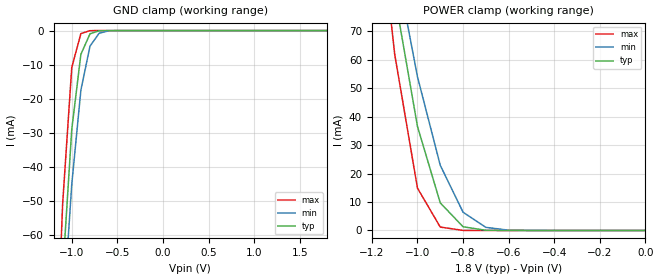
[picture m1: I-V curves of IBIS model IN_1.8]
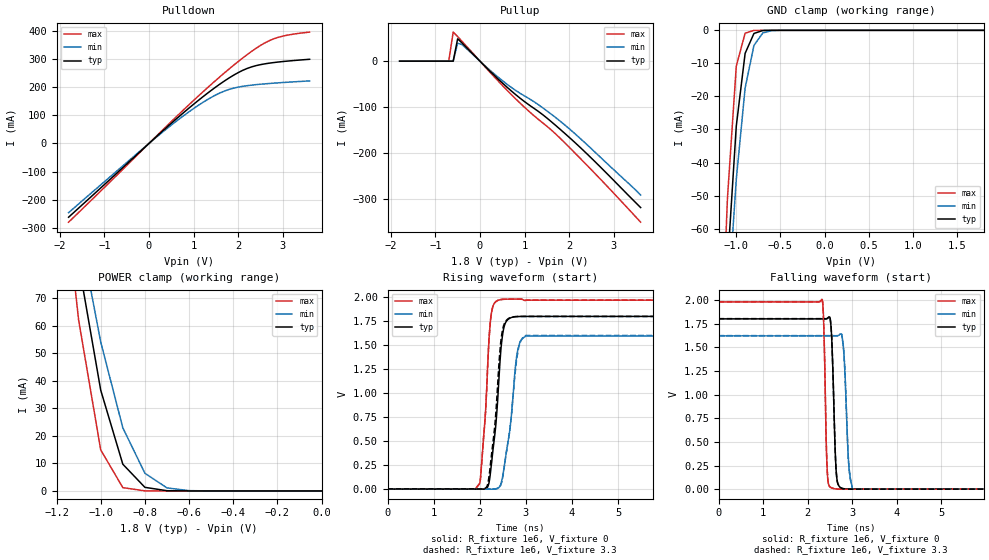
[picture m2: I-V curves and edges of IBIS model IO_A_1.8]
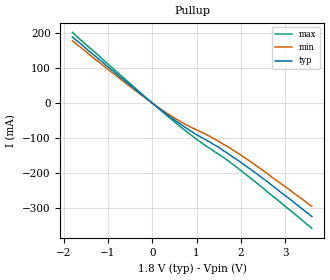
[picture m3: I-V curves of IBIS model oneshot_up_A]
|   DIODES INCORPORATED
|   IBIS Model of PI4ULS3V502
|   Product Family: ULS
|   UQFN (XV) Package
[IBIS Ver] 4.0
[Comment char] |_char
[File Name] pi4uls3v502_xv_reva.ibs
[File Rev] 1.0
[Source] File originated at Diodes Incorporated.
[Date] 10/29/21
[Disclaimer] (C) Copyright DIODES INCORPORATED
   All rights reserved
  Diodes Incorporated hereby grants the user of
  this IBIS model a non-exclusive, nontransferable license to
  use this IBIS model under the following terms.
  This IBIS model is provided on an "AS IS" basis and Diodes
  makes absolutely no warranty with respect to the information
  contained herein. DIODES DISCLAIMS AND CUSTOMER WAIVES ALL
  WARRANTIES, EXPRESSED OR IMPLIED, INCLUDING WARRANTIES OF
  MERCHANTABILITY OR FITNESS FOR A PARTICULAR PURPOSE. The
  entire risk as to quality and performance is with the customer.
  Accordingly, in no event shall the company be liable for any
  damages, whether in contract or tort, including any lost
  profits or other incidental, consequential, exemplary, or
  punitive damages arising out of the use or application of the
  IBIS model provided in this package. Further, Diodes reserves
  the right to make changes without notice to any product herein
  to improve reliability, function, or design. Diodes does not
  convey any license under patent rights or any other intellectual
  property rights, including those of third parties.
  The user is granted this license only to use the IBIS model
  and is not granted rights to sell, load, rent, lease or license
  the IBIS model in whole or in part, or in modified form to anyone
  other than user. User may modify the IBIS model to suit its specific
  application but rights to derivative works and such modifications
  shall belong to Diodes.
  Diodes is not obligated to provide maintenance or support
  for the licensed IBIS model.
  Contact Diodes at ATTN: APPLICATION ENGINEERING / IBIS MODELS
  1545 Barber Ln. Milpitas, CA 95035
[Component] PI4ULS3V502
[Manufacturer] DIODES INCORPORATED
[Package]
| variable   typ   min   max
R_pkg   0.02257ohm   0.02106ohm   0.02498ohm
L_pkg   0.87400nH   0.80200nH   0.98600nH
C_pkg   0.20300pF   0.20050pF   0.20550pF
[Pin] signal_name  model_name   R_pin   L_pin   C_pin
1   VCCA   POWER   0.02498   0.98600n   0.20550p
2   A1   IO_A_1.8   0.02106   0.80200n   0.20050p
3   A2   IO_A_1.8   0.02106   0.80200n   0.20050p
4   GND   GND   0.02498   0.98600n   0.20550p
5   EN   IN_1.8   0.02498   0.98600n   0.20550p
6   B2   IO_B_3.3   0.02106   0.80200n   0.20050p
7   B1   IO_B_3.3   0.02106   0.80200n   0.20050p
8   VCCB   POWER   0.02498   0.98600n   0.20550p
| Models and submodels in the file (9): IN_1.8 (Input), IO_A_1.8 (I/O), oneshot_up_A (Open_source), oneshot_dw_A (Open_sink), 1K_18 (Output), IO_B_3.3 (I/O), oneshot_up_B (Open_source), oneshot_dw_B (Open_sink), 1K_33 (Output)
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|   Model INPUT
[Model]   IN_1.8
Model_type  Input
Vinl=0.54
Vinh=1.26
| variable   typ   min   max
C_comp   1.930pF   1.900pF   1.960pF
[Temperature Range]   25   85   -40
[Voltage range]   1.80V   1.62V   1.98V
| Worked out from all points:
|   GND clamp passes 1 mA (typ) near -0.80 V on its own axis
|   POWER clamp passes 1 mA (typ) near -0.78 V on its own axis
[GND Clamp]
| Voltage   I(typ)   I(min)   I(max)
-1.8V     -540.6mA   -478.5mA   -656.3mA
-1.2V     -126.6mA   -133.1mA   -118.2mA
-1.1V     -71.23mA   -85.2mA    -50.81mA
-1V       -28.95mA   -45.07mA   -10.82mA
-900mV    -6.96mA    -17.47mA   -869.2uA
-800mV    -942.8uA   -4.554mA   -18.94uA
-700mV    -59.43uA   -797.7uA   -152.2nA
-600mV    -1.755uA   -80.71uA   -1.021nA
1.8V      5.4pA      5.981pA    5.4pA
[POWER Clamp]
| Voltage   I(typ)   I(min)   I(max)
-1.8V     557.4mA    486.6mA    695.7mA
-1.2V     140.1mA    144.7mA    134.8mA
-1.1V     82.63mA    96.09mA    62mA
-1V       36.55mA    54.02mA    14.88mA
-900mV    9.698mA    22.9mA     1.197mA
-800mV    1.302mA    6.407mA    22.02uA
-700mV    71.9uA     1.093mA    164.4nA
-600mV    1.944uA    98.92uA    1.069nA
0V        0A         0A         0A
|   Model IO_A
|   Model IO_A_1.8
[Model]   IO_A_1.8
Model_type  I/O
Vinl=0.54
Vinh=1.26
Enable   Active-High
Vref =   0
|Rref =   1000000
|Cref =   0
Vmeas =   0
| variable   typ   min   max
C_comp   8.966pF   8.863pF   9.079pF
[Driver Schedule]
| Model_Name Rise_on_dly Rise_off_dly Fall_on_dly Fall_off_dly
oneshot_up_A   0ns   1.0ns   NA   NA
oneshot_dw_A   NA   NA   0ns   1.0ns
1K_18   0ns   NA   0ns   NA
[Voltage Range]   1.80V   1.62V   1.98V
[POWER Clamp Reference]   1.80V   1.62V   1.98V
[GND Clamp Reference]   0.00V   0.00V   0.00V
[Temperature Range]   25   85   -40
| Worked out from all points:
|   slope of the pulldown table from 0 to 0.27 V, typ, clamps not added: 6.88 ohm
|   slope of the pullup table from 0 to 0.27 V, typ, clamps not added: 10.3 ohm
|   GND clamp passes 1 mA (typ) near -0.80 V on its own axis
|   POWER clamp passes 1 mA (typ) near -0.78 V on its own axis
|   rising waveform, R_fixture 1e6, V_fixture 0: 20-80 % time 181ps typ, 217ps min, 142ps max; typ from 0 V to 1.8 V
|   falling waveform, R_fixture 1e6, V_fixture 0: 20-80 % time 69.4ps typ, 83.1ps min, 53.3ps max; typ from 1.8 V to 0 V
|   rising waveform, R_fixture 1e6, V_fixture 3.3: 20-80 % time 182ps typ, 226ps min, 142ps max; typ from 0.002 V to 1.8 V
|   falling waveform, R_fixture 1e6, V_fixture 3.3: 20-80 % time 69.4ps typ, 83.2ps min, 53.4ps max; typ from 1.8 V to 0 V
[GND Clamp]
| Voltage   I(typ)   I(min)   I(max)
-1.8V     -540.6mA   -478.5mA   -656.3mA
-1.2V     -126.6mA   -133.1mA   -118.2mA
-1.1V     -71.23mA   -85.2mA    -50.81mA
-1V       -28.95mA   -45.07mA   -10.82mA
-900mV    -6.96mA    -17.47mA   -869.2uA
-800mV    -942.8uA   -4.554mA   -18.94uA
-700mV    -59.43uA   -797.7uA   -152.2nA
-600mV    -1.755uA   -80.71uA   -1.021nA
1.8V      5.4pA      5.981pA    5.4pA
[POWER Clamp]
| Voltage   I(typ)   I(min)   I(max)
-1.8V     557.4mA    486.6mA    695.7mA
-1.2V     140.1mA    144.7mA    134.8mA
-1.1V     82.63mA    96.09mA    62mA
-1V       36.55mA    54.02mA    14.88mA
-900mV    9.698mA    22.9mA     1.197mA
-800mV    1.302mA    6.407mA    22.02uA
-700mV    71.9uA     1.093mA    164.4nA
-600mV    1.944uA    98.92uA    1.069nA
0V        0A         0A         0A
[Pulldown]
| Voltage   I(typ)   I(min)   I(max)
-1.8V     -262.9mA   -246.7mA   -280.6mA
400mV     57.82mA    52.72mA    62.58mA
900mV     126.6mA    113.4mA    138.6mA
1.4V      189.9mA    164.7mA    211.3mA
1.7V      223.8mA    187.6mA    252.9mA
2.1V      260.8mA    203.8mA    304.7mA
2.3V      273.2mA    208.1mA    328.4mA
2.6V      284.1mA    212.7mA    358.9mA
2.8V      288.7mA    215.2mA    373.5mA
3V        292.2mA    217.4mA    382.8mA
3.6V      300.3mA    223.2mA    397.3mA
[Pullup]
| Voltage   I(typ)   I(min)   I(max)
-1.8V     3.473nA    72nA       347.7pA
-700mV    1.934nA    41.34nA    217.4pA
-600mV    43.57nA    43.73nA    63.41mA
-500mV    48.75mA    39.12mA    53.6mA
-400mV    39.49mA    36.01mA    43.02mA
200mV     -19.58mA   -17.72mA   -21.67mA
600mV     -56.22mA   -49.87mA   -62.71mA
900mV     -80.85mA   -70.11mA   -91.58mA
1.3V      -109mA     -94.33mA   -126.3mA
1.9V      -157.5mA   -139.1mA   -178mA
2.5V      -211.9mA   -191.3mA   -237.3mA
3.6V      -319.3mA   -292.1mA   -351.2mA
[Rising Waveform]
| IO_33
R_fixture =   1e6
C_fixture =   0
L_fixture =   0
V_fixture =   0
V_fixture_min = 0
V_fixture_max = 0
|   Time   V(typ)   V(min)   V(max)
0s        93.22uV    181.2uV    45.47uV
2ns       -76.7uV    166uV      58.96mV
2.125ns   4.334mV    178.3uV    808.9mV
2.237ns   196.6mV    -214.7uV   1.782V
2.4ns     1.029V     12.09mV    1.969V
2.462ns   1.479V     61.09mV    1.976V
2.55ns    1.727V     299.5mV    1.979V
2.8ns     1.798V     1.386V     1.98V
3ns       1.8V       1.595V     1.97V
12ns      1.8V       1.595V     1.97V
[Falling Waveform]
| IO_33
R_fixture =   1e6
C_fixture =   0
L_fixture =   0
V_fixture =   0
V_fixture_min = 0
V_fixture_max = 0
|   Time   V(typ)   V(min)   V(max)
0s        1.8V       1.621V     1.979V
2.325ns   1.8V       1.621V     2.005V
2.362ns   1.8V       1.621V     1.697V
2.438ns   1.803V     1.621V     192.3mV
2.55ns    1.454V     1.62V      11.21mV
2.662ns   83.92mV    1.621V     1.929mV
2.8ns     5.453mV    1.505V     330.9uV
2.912ns   1.127mV    316.4mV    144.7uV
3ns       419.6uV    343.1uV    914.7uV
12ns      419.6uV    343.1uV    914.7uV
[Rising Waveform]
| IO_33
R_fixture =   1e6
C_fixture =   0
L_fixture =   0
V_fixture =   3.3
V_fixture_min = 3
V_fixture_max = 3.6
|   Time   V(typ)   V(min)   V(max)
0s        2.151mV    2.103mV    2.239mV
2ns       1.833mV    2.085mV    60.68mV
2.162ns   36.19mV    2.068mV    1.185V
2.237ns   285.8mV    1.762mV    1.782V
2.4ns     1.19V      11.52mV    1.969V
2.462ns   1.562V     54.55mV    1.976V
2.537ns   1.73V      253mV      1.979V
2.8ns     1.799V     1.357V     1.98V
3ns       1.8V       1.602V     1.97V
12ns      1.8V       1.602V     1.97V
[Falling Waveform]
| IO_33
R_fixture =   1e6
C_fixture =   0
L_fixture =   0
V_fixture =   3.3
V_fixture_min = 3
V_fixture_max = 3.6
|   Time   V(typ)   V(min)   V(max)
0s        1.802V     1.623V     1.982V
2.325ns   1.802V     1.623V     2.007V
2.362ns   1.802V     1.623V     1.699V
2.438ns   1.805V     1.623V     192.9mV
2.55ns    1.456V     1.623V     11.24mV
2.662ns   84.2mV     1.623V     1.986mV
2.8ns     5.476mV    1.513V     372.2uV
2.912ns   1.142mV    322mV      163.9uV
3ns       432.9uV    344.2uV    1.001mV
12ns      432.9uV    344.2uV    1.001mV
[Ramp]
| variable   typ   min   max
dV/dt_r   1.08/185.14E-12   1.296/229.51E-12   1.568/148.07E-12
dV/dt_f   1.08/64.391E-12   1.296/81.134E-12   1.568/51.782E-12
R_load = 1.00E+6
[Model]   oneshot_up_A
Model_type  Open_source
Vref = 0
Rref = 50
Vmeas = 0.9
C_comp   8.966pF   8.863pF   9.079pF
[Voltage Range]   1.80V   1.62V   1.98V
[Temperature Range]   25   85   -40
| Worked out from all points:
|   slope of the pullup table from 0 to 0.27 V, typ, clamps not added: 10.2 ohm
[Pullup]
-1.8V     188mA      177mA      201mA
-600mV    61.5mA     56.8mA     66.4mA
200mV     -19.7mA    -17.8mA    -21.7mA
600mV     -56.9mA    -50mA      -63.7mA
1V        -89.9mA    -76.4mA    -103mA
1.5V      -126mA     -109mA     -146mA
2V        -169mA     -148mA     -192mA
2.6V      -224mA     -201mA     -253mA
3.6V      -323mA     -294mA     -356mA
[Ramp]
| variable   typ   min   max
dV/dt_r   0.89/176.8E-12   0.78/224.6E-12   1.00/138.6E-12
dV/dt_f   0.89/444.5E-12   0.78/435.1E-12   1.00/446.5E-12
R_load = 50
